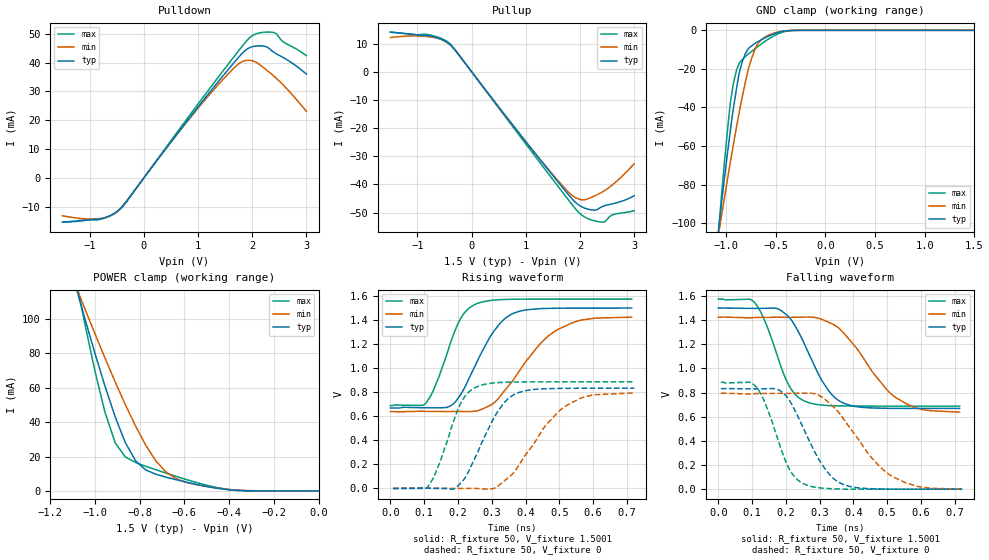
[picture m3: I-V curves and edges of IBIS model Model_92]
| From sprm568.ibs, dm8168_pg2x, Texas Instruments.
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| Model based on original model for BSHTLTCSCDVGPBFZ
|   Sub model FAST_10MA_5PER_1P5
[model]   Model_92
|[Description]  [1.5V-3-STATE-X-FAST:10MA, IND, 5%]
|   Fast slew rate (SR[1:0] = "10"), 0.80 * RExt = 1.250 * Iout
|   (I[2:0] = "101"), 10mA nominal with Rext = 50R, ,Industrial
|   temperature range (-40C to 125C, 25C nominal),5% power supply
|   tolerance
|[Input Load]
|[Output Drive] FAST:10MA
|Voltage   1.5V
|Mode   3-STATE
Model_type   3-state
Polarity   Non-Inverting
Enable   Active-Low
Cref =  15.0000pF
Rref =  100.0000M
Vref =  0V
Vmeas =  0.75005
C_comp   1.5249p   1.4275p   1.6205p
[Model Spec]
[Temperature Range]   25   125   -40
[Voltage Range]   1.5   1.425   1.575
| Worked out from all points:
|   slope of the pulldown table from 0 to 0.225 V, typ, clamps not added: 39.9 ohm
|   slope of the pullup table from 0 to 0.225 V, typ, clamps not added: 39.8 ohm
|   GND clamp passes 1 mA (typ) near -0.47 V on its own axis
|   POWER clamp passes 1 mA (typ) near -0.42 V on its own axis
|   rising waveform, R_fixture 50, V_fixture 1.5001: 20-80 % time 94.2ps typ, 134ps min, 70.4ps max; typ from 0.669 V to 1.5 V
|   rising waveform, R_fixture 50, V_fixture 0: 20-80 % time 89ps typ, 124ps min, 67.7ps max; typ from 0 V to 0.834 V
|   falling waveform, R_fixture 50, V_fixture 1.5001: 20-80 % time 90.7ps typ, 130ps min, 71ps max; typ from 1.5 V to 0.669 V
|   falling waveform, R_fixture 50, V_fixture 0: 20-80 % time 92.1ps typ, 132ps min, 69ps max; typ from 0.833 V to 0 V
[POWER_clamp]
-1.5V     321.7mA    260.6mA    415.9mA
-1.076V   114.2mA    115.8mA    116.9mA
-1.061V   107.2mA    110.9mA    107.1mA
-954.6mV  60.59mA    77.06mA    45.35mA
-909.2mV  42.85mA    63.21mA    27.81mA
-863.7mV  27.9mA     49.99mA    19.69mA
-818.2mV  17.49mA    37.63mA    16.52mA
-772.8mV  12.19mA    26.53mA    14.33mA
-681.9mV  7.985mA    10.89mA    10.33mA
-590.9mV  5.094mA    4.955mA    6.6mA
-363.7mV  298.5uA    465.2uA    297.6uA
0V        1.518nA    24.08nA    367.8pA
[Pulldown]
-1.5V     -15.29mA   -13.07mA   -15.28mA
-772.8mV  -14.07mA   -13.9mA    -14.11mA
-590.9mV  -12.74mA   -12.86mA   -12.82mA
-409.1mV  -10.08mA   -10.11mA   -10.32mA
1.046V    25.68mA    25.17mA    26.75mA
1.591V    38.31mA    36.75mA    40.25mA
1.818V    43.24mA    40.36mA    45.69mA
1.955V    45.18mA    40.77mA    48.64mA
2.091V    45.77mA    39.91mA    50.06mA
2.273V    45.4mA     37.32mA    50.56mA
2.364V    44.07mA    35.93mA    50.51mA
3V        36.04mA    23.14mA    42.4mA
[Pullup]
-1.5V     14.1mA     12.18mA    14.13mA
-818.2mV  12.87mA    12.54mA    13.29mA
-590.9mV  11.83mA    11.72mA    12.11mA
-409.1mV  9.844mA    9.773mA    10.15mA
1.227V    -30.36mA   -30.27mA   -31.43mA
1.727V    -42.29mA   -41.55mA   -44.05mA
1.909V    -46.29mA   -44.65mA   -48.54mA
2.046V    -48.11mA   -45.48mA   -51.1mA
2.227V    -49.12mA   -44.44mA   -52.74mA
2.409V    -47.87mA   -42.71mA   -53.43mA
2.591V    -46.92mA   -40.26mA   -50.87mA
3V        -44.02mA   -32.61mA   -49.35mA
[GND_clamp]
-1.5V     -310.1mA   -250.5mA   -402.5mA
-1.076V   -103.6mA   -106.2mA   -105.2mA
-1.046V   -89.81mA   -96.36mA   -86.02mA
-954.6mV  -51.22mA   -67.87mA   -36.88mA
-924.3mV  -40.08mA   -58.86mA   -27.29mA
-863.7mV  -21.24mA   -41.56mA   -16.73mA
-833.4mV  -15.8mA    -33.75mA   -15.03mA
-772.8mV  -9.345mA   -19.75mA   -12.19mA
-712.2mV  -6.928mA   -10.35mA   -9.704mA
-621.3mV  -4.261mA   -3.896mA   -6.225mA
-409.1mV  -337.1uA   -289.1uA   -618.9uA
1.5V      1.518nA    257.2nA    299pA
[Ramp]
dV/dt_f   0.665384/0.13628682n   0.629864/0.2000188n   0.71/0.10897595n
dV/dt_r  0.6716992/0.13165568n 0.64196624/0.19536277n 0.71221096/0.10400915n
R_load = 50
[Rising Waveform]
R_fixture = 50
V_fixture = 1.5001
V_fixture_min = 1.425
V_fixture_max = 1.575
0s        669.3mV    639.1mV    688.4mV
105.5ps   671.2mV    640.7mV    711.5mV
142.2ps   670.7mV    640mV      918.4mV
185ps     700.3mV    640mV      1.266V
216.8ps   823.1mV    639.6mV    1.451V
252.2ps   1.029V     643.2mV    1.533V
305.6ps   1.305V     709.3mV    1.566V
365.1ps   1.458V     907.7mV    1.574V
493.9ps   1.499V     1.319V     1.575V
714.3ps   1.5V       1.425V     1.575V
[Rising Waveform]
R_fixture = 50
V_fixture = 0
V_fixture_min = 0
V_fixture_max = 0
7.64ps    0V         0V         0V
110.5ps   2.343mV    2.194mV    13.95mV
145.4ps   0V         0V         210.2mV
191.2ps   0V         0V         591.8mV
250.5ps   253.8mV    0V         838.4mV
315.4ps   629.3mV    13.46mV    879.7mV
376ps     792.9mV    173.4mV    885.4mV
459ps     829.1mV    521.5mV    886.6mV
523.4ps   832.6mV    693.5mV    886.7mV
721.9ps   833.5mV    794.6mV    886.9mV
[Falling Waveform]
R_fixture = 50
V_fixture = 1.5001
V_fixture_min = 1.425
V_fixture_max = 1.575
0s        1.499V     1.424V     1.575V
110ps     1.497V     1.422V     1.537V
186ps     1.479V     1.424V     1.012V
215.1ps   1.405V     1.423V     830.6mV
252.6ps   1.216V     1.425V     732.6mV
322.7ps   831mV      1.387V     693mV
371.6ps   711.6mV    1.292V     689mV
521.6ps   669.3mV    766.3mV    687.8mV
591.8ps   668.8mV    667.7mV    687.7mV
714.3ps   668.6mV    638.2mV    687.6mV
[Falling Waveform]
R_fixture = 50
V_fixture = 0
V_fixture_min = 0
V_fixture_max = 0
7.64ps    832.6mV    794mV      886mV
114.7ps   830.5mV    791.9mV    840.4mV
190.7ps   800.2mV    793.4mV    294.1mV
217.4ps   702.7mV    792.9mV    133.3mV
249.8ps   516.9mV    794.7mV    48.09mV
316.2ps   167mV      742.5mV    6.486mV
374.6ps   33.88mV    566mV      0V
458.7ps   3.338mV    244.1mV    0V
518.2ps   0V         100.8mV    0V
721.9ps   0V         0V         0V
